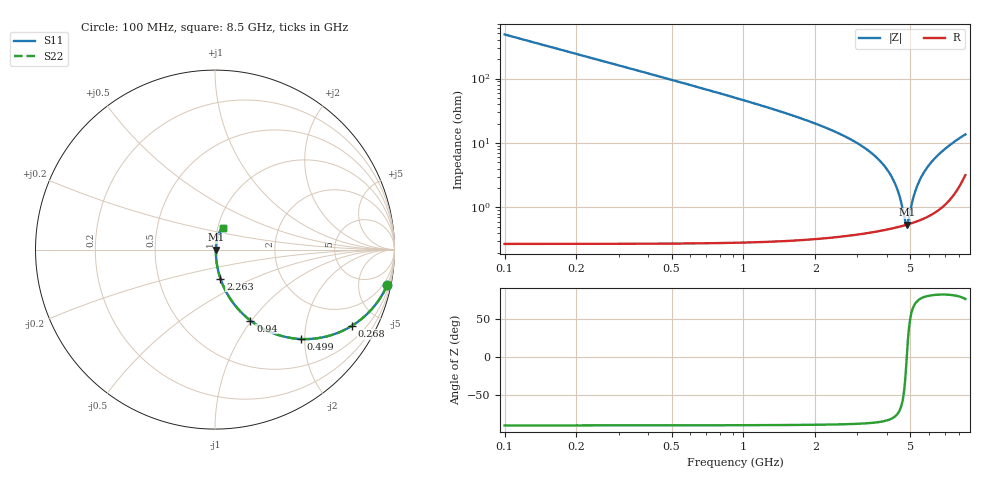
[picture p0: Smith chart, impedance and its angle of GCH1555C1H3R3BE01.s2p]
!Murata Part Number: GCH1555C1H3R3BE01
!These Parameters are Measured in Series Mode Connection
!Data Generated on Mar 13, 2026
!  o--ll--o
!Port1  Port2
!  o------o
!Operation Temp=25[degC], DC Bias Voltage=0[V]
!Freq. Start=100[MHz] Stop=9[GHz] 401[Steps]
# Hz S RI R 50
!Freq.(Hz) S11(Real) S11(Imag) S21(Real) S21(Imag) S12(Real) S12(Imag) S22(Real) S22(Imag)
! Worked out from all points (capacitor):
!   401 points, 100 MHz to 8.5 GHz, reference 50 ohm
!   read as one part in series: C = 3.3 pF near 142 MHz
!   lowest |Z| = 540 mohm at 4.825 GHz (marker M1)
!   series resonance near 4.829 GHz, so ESL is about 330 pH
!   S11 on the Smith chart (normalised r, x): 100 MHz: 1.01, -9.64; 268 MHz: 1.01, -3.59; 499 MHz: 1.01, -1.91; 940 MHz: 1.01, -0.99; 2.263 GHz: 1.01, -0.33; 8.5 GHz: 1.06, +0.26
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1e8  0.9586 -0.1988  0.0414 0.1988  0.0414 0.1988  0.9586 -0.1988
2.05e8  0.8462 -0.3602  0.1538 0.3602  0.1538 0.3602  0.8462 -0.3602
2.68e8  0.7626 -0.4247  0.2374 0.4247  0.2374 0.4247  0.7626 -0.4247
3.73e8  0.6227 -0.4836  0.3773 0.4836  0.3773 0.4836  0.6227 -0.4836
4.99e8  0.4777 -0.4981  0.5223 0.4981  0.5223 0.4981  0.4777 -0.4981
7.09e8  0.3078 -0.4595  0.6922 0.4595  0.6922 0.4595  0.3078 -0.4595
9.4e8  0.1974 -0.3952  0.8026 0.3952  0.8026 0.3952  0.1974 -0.3952
1.507e9  0.0795 -0.2654  0.9205 0.2654  0.9205 0.2654  0.0795 -0.2654
2.263e9  0.0301 -0.1612  0.9699 0.1612  0.9699 0.1612  0.0301 -0.1612
2.914e9  0.0147 -0.1038  0.9853 0.1038  0.9853 0.1038  0.0147 -0.1038
3.754e9  0.00692 -0.0507  0.9931 0.0507  0.9931 0.0507  0.00692 -0.0507
4.3e9  0.00535 -0.0233  0.9946 0.0233  0.9946 0.0233  0.00535 -0.0233
4.51e9  0.0052 -0.0137  0.9948 0.0137  0.9948 0.0137  0.0052 -0.0137
4.762e9  0.0053 -0.00282  0.9947 0.00282  0.9947 0.00282  0.0053 -0.00282
4.825e9  0.00537 -0.000176  0.9946 0.000176  0.9946 0.000176  0.00537 -0.000176
4.888e9  0.00545 0.00244  0.9946 -0.00244  0.9946 -0.00244  0.00545 0.00244
5.077e9  0.00579 0.0101  0.9942 -0.0101  0.9942 -0.0101  0.00579 0.0101
5.245e9  0.00621 0.0167  0.9938 -0.0167  0.9938 -0.0167  0.00621 0.0167
5.707e9  0.00788 0.0341  0.9921 -0.0341  0.9921 -0.0341  0.00788 0.0341
6.295e9  0.0112 0.055  0.9888 -0.055  0.9888 -0.055  0.0112 0.055
7.114e9  0.0185 0.0824  0.9815 -0.0824  0.9815 -0.0824  0.0185 0.0824
8.5e9  0.0464 0.122  0.9536 -0.122  0.9536 -0.122  0.0464 0.122
